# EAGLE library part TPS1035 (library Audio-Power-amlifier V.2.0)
TPS1035 is a MONO ended 20W continuous average power per channel, Class-T Digital Audio Power A m p l i f i e r u s i n g T r i p a t h ’ s p r o p r i e t a r y D i g i t a l P o w e r P r o c e s s i n gT M t e c h n o l o g y .
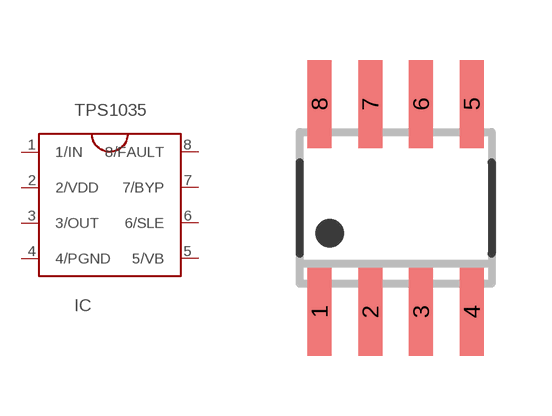
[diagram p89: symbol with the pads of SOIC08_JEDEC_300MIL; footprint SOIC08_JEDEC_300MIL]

Designator prefix IC

## TPS1035  [SOIC08_JEDEC_300MIL]
1  1/IN
2  2/VDD  pwr
3  3/OUT  out
4  4/PGND  pwr
5  5/VB
6  6/SLE
7  7/BYP
8  8/FAULT

## Footprint SOIC08_JEDEC_300MIL (pad centres in mm)
SOIC 08 JEDEC 150mil Small Outline Narrow Plastic Gull Wing 150-mil body, package type SN
smd 0.6 x 2.2: 1 -1.905,-2.6; 2 -0.635,-2.6; 3 0.635,-2.6; 4 1.905,-2.6; 5 1.905,2.6; 6 0.635,2.6; 7 -0.635,2.6; 8 -1.905,2.6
